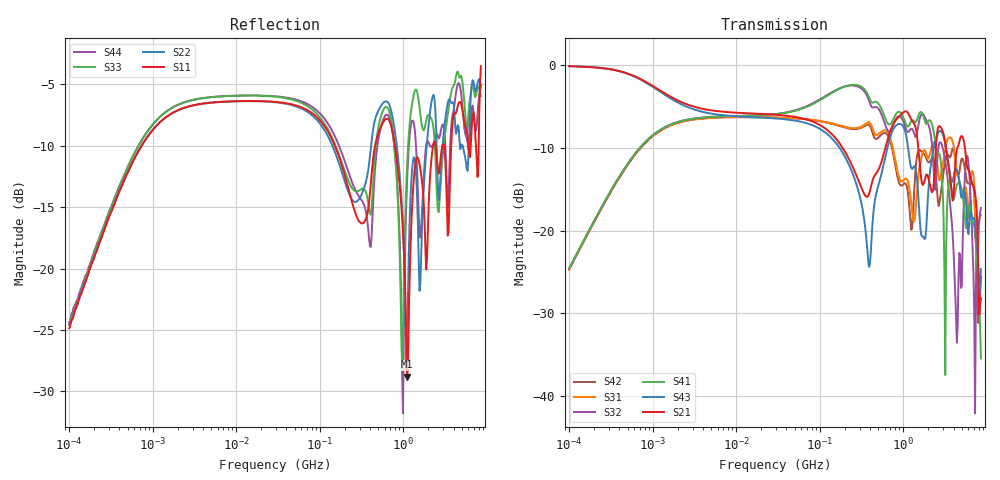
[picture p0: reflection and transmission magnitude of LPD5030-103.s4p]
# MHz S MA R 50
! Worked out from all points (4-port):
!   498 points, 100 kHz to 8.5 GHz, reference 50 ohm
!   strongest paths, dB at 100 kHz, 1.698 MHz, 29.49 MHz, 500.7 MHz, 8.5 GHz:
!     S21: -0.1, -3.9, -6.0, -12.7, -28.2
!     S43: -0.1, -4.1, -6.4, -14.6, -24.7
!     S41: -24.6, -7.1, -5.9, -4.6, -35.5
!     S32: -24.6, -7.1, -5.9, -5.2, -17.3
!     S31: -24.7, -7.2, -6.3, -8.4, -18.1
!     S42: -24.7, -7.2, -6.3, -8.8, -25.6
!   lowest |S11| = -28.8 dB at 1.113 GHz (marker M1), VSWR 1.08, Z = 52.7 + j2.57 ohm
!   |S11| at or under -10 dB: 796.1 MHz to 2.279 GHz (1.483 GHz wide, 96.4 % of centre); 2.441 GHz to 2.946 GHz (504.5 MHz wide, 18.7 % of centre); 3.067 GHz to 3.753 GHz (686.8 MHz wide, 20.1 % of centre)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
0.1  0.05708 81.3  0.9873 -3.3  0.05795 -97.6  0.05914 82.5
     0.9873 -3.3  0.05916 81.4  0.0588 82.7  0.05815 -97.9
     0.05795 -97.6  0.0588 82.7  0.05889 81.4  0.988 -3.5
     0.05914 82.5  0.05815 -97.9  0.988 -3.5  0.06034 83.0
179.1505  0.2711 -58.3  0.3285 -90.2  0.4307 78.3  0.7278 -21.0
          0.3285 -90.2  0.2539 -50.1  0.7312 -23.5  0.427 79.5
          0.4307 78.3  0.7312 -23.5  0.2772 -52.1  0.3083 -93.6
          0.7278 -21.0  0.427 79.5  0.3083 -93.6  0.3024 -56.4
673.7244  0.4022 -113.7  0.3786 30.5  0.3813 -91.4  0.4384 -110.5
          0.3786 30.5  0.4683 -109.8  0.397 -112.5  0.3648 -89.1
          0.3813 -91.4  0.397 -112.5  0.4398 -104.3  0.3453 34.0
          0.4384 -110.5  0.3648 -89.1  0.3453 34.0  0.4154 -109.9
1113.489  0.03624 42.3  0.5224 -114.1  0.2036 172.5  0.4273 -171.3
          0.5224 -114.1  0.04318 -125.3  0.3979 -175.0  0.1815 168.3
          0.2036 172.5  0.3979 -175.0  0.2647 -84.7  0.3487 -137.5
          0.4273 -171.3  0.1815 168.3  0.3487 -137.5  0.231 -81.3
3183.684  0.2772 -70.0  0.3387 -66.8  0.3122 -35.4  0.01339 22.5
          0.3387 -66.8  0.4047 -25.4  0.2639 -142.2  0.2645 -35.5
          0.3122 -35.4  0.2639 -142.2  0.3571 -23.4  0.334 -64.4
          0.01339 22.5  0.2645 -35.5  0.334 -64.4  0.3226 -69.4
4588.001  0.4708 -171.9  0.3286 135.4  0.208 94.2  0.1952 96.0
          0.3286 135.4  0.3792 169.5  0.05196 -140.0  0.2171 108.8
          0.208 94.2  0.05196 -140.0  0.6198 161.4  0.2165 105.0
          0.1952 96.0  0.2171 108.8  0.2165 105.0  0.57 -179.8
8500  0.6673 -15.2  0.03887 -128.7  0.1238 -19.7  0.01687 26.6
      0.03887 -128.7  0.5541 -49.7  0.1372 42.1  0.05273 5.4
      0.1238 -19.7  0.1372 42.1  0.5041 -55.7  0.05852 -7.0
      0.01687 26.6  0.05273 5.4  0.05852 -7.0  0.5547 -36.2
